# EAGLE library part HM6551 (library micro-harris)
MICROCONTROLLER/MEMORY DEVICE
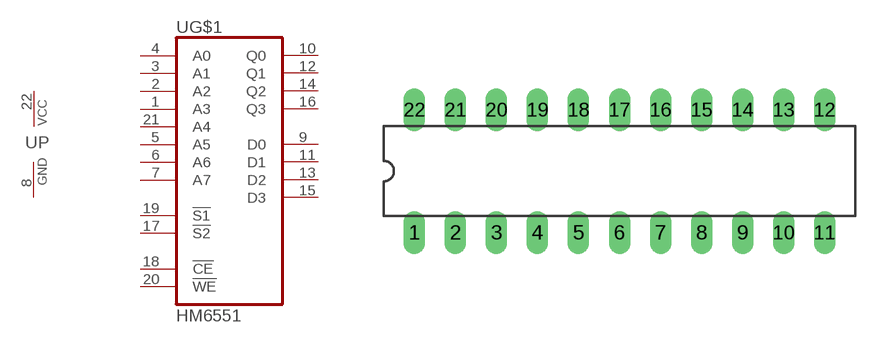
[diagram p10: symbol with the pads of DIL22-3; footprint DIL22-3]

Designator prefix U; gates G$1=HM6551 P=PWRN

## HM6551 (OC_FARNELL: unknown; OC_NEWARK: unknown)  [DIL22-3]
1  G$1:A3  in
2  G$1:A2  in
3  G$1:A1  in
4  G$1:A0  in
5  G$1:A5  in
6  G$1:A6  in
7  G$1:A7  in
8  P:GND  pwr
9  G$1:D0  in
10  G$1:Q0  hiz
11  G$1:D1  in
12  G$1:Q1  hiz
13  G$1:D2  in
14  G$1:Q2  hiz
15  G$1:D3  in
16  G$1:Q3  hiz
17  G$1:!S2  in
18  G$1:!CE  in
19  G$1:!S1  in
20  G$1:!WE  in
21  G$1:A4  in
22  P:VCC  pwr

## Footprint DIL22-3 (pad centres in mm)
Dual In Line Package 0.3 inch
drill 0.813 long: 1 -12.7,-3.81; 2 -10.16,-3.81; 3 -7.62,-3.81; 4 -5.08,-3.81; 5 -2.54,-3.81; 6 0,-3.81; 7 2.54,-3.81; 8 5.08,-3.81; 9 7.62,-3.81; 10 10.16,-3.81; 11 12.7,-3.81; 12 12.7,3.81; 13 10.16,3.81; 14 7.62,3.81; 15 5.08,3.81; 16 2.54,3.81; 17 0,3.81; 18 -2.54,3.81; 19 -5.08,3.81; 20 -7.62,3.81; 21 -10.16,3.81; 22 -12.7,3.81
